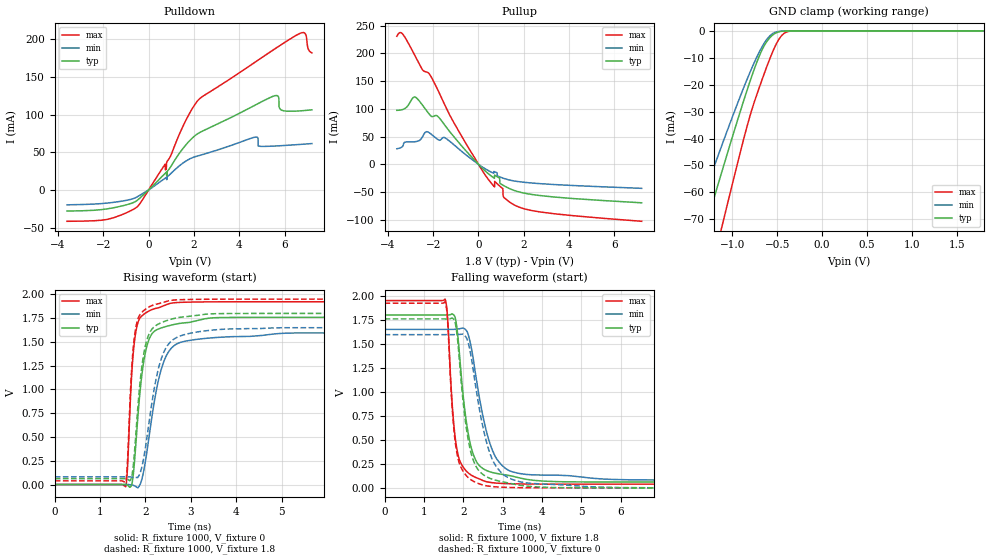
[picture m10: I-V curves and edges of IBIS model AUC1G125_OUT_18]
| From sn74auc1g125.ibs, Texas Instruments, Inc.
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[Model]   AUC1G125_OUT_18
Model_type  3-state
Enable   Active-Low
Vref =   0
Rref =   1000
Cref =   30p
Vmeas =   0.9
| variable   typ   min   max
C_comp   7.42pF   5.09pF   18.55pF
| C_pullup   6.33pF   3.20pF   11.74pF
| C_pulldown   9.19pF   5.45pF   19.79pF
| C_tri-state   7.42pF   5.09pF   18.55pF
[Temperature Range]   40   100   -40
| Ambient temperature   25   85   -40
[Voltage range]   1.8   1.65   1.95
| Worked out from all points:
|   slope of the pulldown table from 0 to 0.27 V, typ, clamps not added: 34.4 ohm
|   slope of the pullup table from 0 to 0.27 V, typ, clamps not added: 24.6 ohm
|   GND clamp passes 1 mA (typ) near -0.53 V on its own axis
|   rising waveform, R_fixture 1000, V_fixture 0: 20-80 % time 230ps typ, 368ps min, 142ps max; typ from 0 V to 1.76 V
|   falling waveform, R_fixture 1000, V_fixture 1.8: 20-80 % time 318ps typ, 481ps min, 201ps max; typ from 1.8 V to 0.061 V
|   rising waveform, R_fixture 1000, V_fixture 1.8: 20-80 % time 225ps typ, 357ps min, 140ps max; typ from 0.061 V to 1.8 V
|   falling waveform, R_fixture 1000, V_fixture 0: 20-80 % time 320ps typ, 478ps min, 201ps max; typ from 1.76 V to 0 V
[GND Clamp]
| AUC1G125_OUT_18
|   Voltage   I(typ)   I(min)   I(max)
-3.6V     -338.8mA   -286.3mA   -409.7mA
-1.44V    -88.88mA   -72.66mA   -117.1mA
-1.285V   -71.24mA   -58.05mA   -95.84mA
-1.14V    -54.92mA   -44.63mA   -75.98mA
-1.095V   -49.91mA   -40.54mA   -69.84mA
-840mV    -22.47mA   -18.35mA   -35.96mA
-695mV    -8.981mA   -7.553mA   -20.59mA
-575mV    -2.299mA   -1.652mA   -9.733mA
-490mV    -465.5uA   -257.7uA   -3.617mA
-425mV    -91.45uA   -52.83uA   -990.1uA
-275mV    -1.057uA   -972.3nA   -6.251uA
1.8V      429.2pA    31.06nA    480.6pA
[Pulldown]
| AUC1G125_OUT_18
|   Voltage   I(typ)   I(min)   I(max)
-3.6V     -28.02mA   -19.77mA   -41.61mA
-570mV    -15.18mA   -10.2mA    -23.87mA
780mV     23.41mA    16.52mA    27.8mA
1.53V     55.61mA    35.96mA    85.47mA
2.26V     76.24mA    45.87mA    121.3mA
4.705V    112.6mA    70.03mA    169.6mA
4.835V    114.6mA    58.3mA     172.3mA
5.575V    125mA      58.22mA    187.2mA
5.845V    106.1mA    58.68mA    192.6mA
6.69V     104.8mA    60.37mA    207.8mA
6.915V    105.4mA    60.85mA    206.9mA
7.2V      106.2mA    61.47mA    181.7mA
[Pullup]
| AUC1G125_OUT_18
|   Voltage   I(typ)   I(min)   I(max)
-3.6V     97.21mA    27.98mA    230.6mA
-3.35V    98.65mA    32.03mA    234.9mA
-2.755V   120.2mA    40.97mA    192.2mA
-2.295V   97.07mA    58.73mA    166.3mA
-1.495V   71.17mA    48.15mA    108mA
225mV     -9.265mA   -6.217mA   -14.9mA
710mV     -19.38mA   -13.4mA    -40.76mA
1.075V    -37.42mA   -24.78mA   -43.8mA
1.095V    -37.9mA    -25.06mA   -57.63mA
1.31V     -42.56mA   -27.71mA   -66.07mA
2.685V    -56.12mA   -34.74mA   -85.59mA
7.2V      -69.32mA   -43.26mA   -102.6mA
[Ramp]
| AUC1G125_OUT_18
| variable   typ   min   max
dV/dt_r   1.07/2.36E-10   0.98/3.77E-10   1.17/1.44E-10
dV/dt_f   1.05/3.18E-10   0.95/4.90E-10   1.16/2.02E-10
R_load = 1000
[Rising Waveform]
| AUC1G125_OUT_18
R_fixture =   1000
C_fixture =   0
L_fixture =   0
V_fixture =   0
V_fixture_min = 0
V_fixture_max = 0
|   Time   V(typ)   V(min)   V(max)
0s        6.96nV     23.5nV     1.103nV
1.565ns   -843.3uV   556.2uV    -23.88mV
1.605ns   -6.937mV   691.5uV    189.3mV
1.705ns   16.38mV    -5.023mV   1.223V
1.82ns    634.9mV    -31.46mV   1.68V
1.935ns   1.208V     83.65mV    1.78V
2.07ns    1.515V     471.3mV    1.823V
2.32ns    1.642V     1.163V     1.864V
2.605ns   1.681V     1.45V      1.91V
29.99ns   1.759V     1.595V     1.923V
[Falling Waveform]
| AUC1G125_OUT_18
R_fixture =   1000
C_fixture =   0
L_fixture =   0
V_fixture =   1.8
V_fixture_min = 1.65
V_fixture_max = 1.95
|   Time   V(typ)   V(min)   V(max)
0s        1.8V       1.65V      1.95V
1.54ns    1.8V       1.65V      1.964V
1.6ns     1.8V       1.65V      1.786V
1.75ns    1.804V     1.65V      709.4mV
1.88ns    1.507V     1.655V     324.9mV
2.195ns   431.1mV    1.48V      134.9mV
2.69ns    165.5mV    449mV      56.59mV
3.245ns   122.2mV    167mV      42.06mV
5.825ns   60.83mV    87.15mV    38.59mV
29.99ns   61.05mV    81.2mV     38.68mV
[Rising Waveform]
| AUC1G125_OUT_18
R_fixture =   1000
C_fixture =   0
L_fixture =   0
V_fixture =   1.8
V_fixture_min = 1.65
V_fixture_max = 1.95
|   Time   V(typ)   V(min)   V(max)
0s        61.05mV    81.2mV     38.68mV
1.565ns   60.3mV     81.56mV    25.35mV
1.6ns     56.79mV    81.63mV    206.3mV
1.7ns     89.08mV    78.16mV    1.248V
1.81ns    673.9mV    74.02mV    1.703V
1.92ns    1.239V     184.4mV    1.811V
2.045ns   1.541V     538.7mV    1.858V
2.29ns    1.689V     1.227V     1.903V
2.57ns    1.739V     1.508V     1.938V
29.99ns   1.8V       1.65V      1.95V
[Falling Waveform]
| AUC1G125_OUT_18
R_fixture =   1000
C_fixture =   0
L_fixture =   0
V_fixture =   0
V_fixture_min = 0
V_fixture_max = 0
|   Time   V(typ)   V(min)   V(max)
0s        1.759V     1.595V     1.923V
1.54ns    1.759V     1.595V     1.935V
1.6ns     1.759V     1.595V     1.751V
1.745ns   1.76V      1.595V     692.1mV
1.865ns   1.508V     1.597V     310.4mV
2.165ns   420.3mV    1.444V     93.3mV
2.605ns   113mV      456.3mV    20.41mV
3.25ns    41.94mV    87.03mV    3.426mV
5.375ns   34.86uV    9.189mV    -131.8uV
29.99ns   3.105uV    -1.033uV   338.8nV
